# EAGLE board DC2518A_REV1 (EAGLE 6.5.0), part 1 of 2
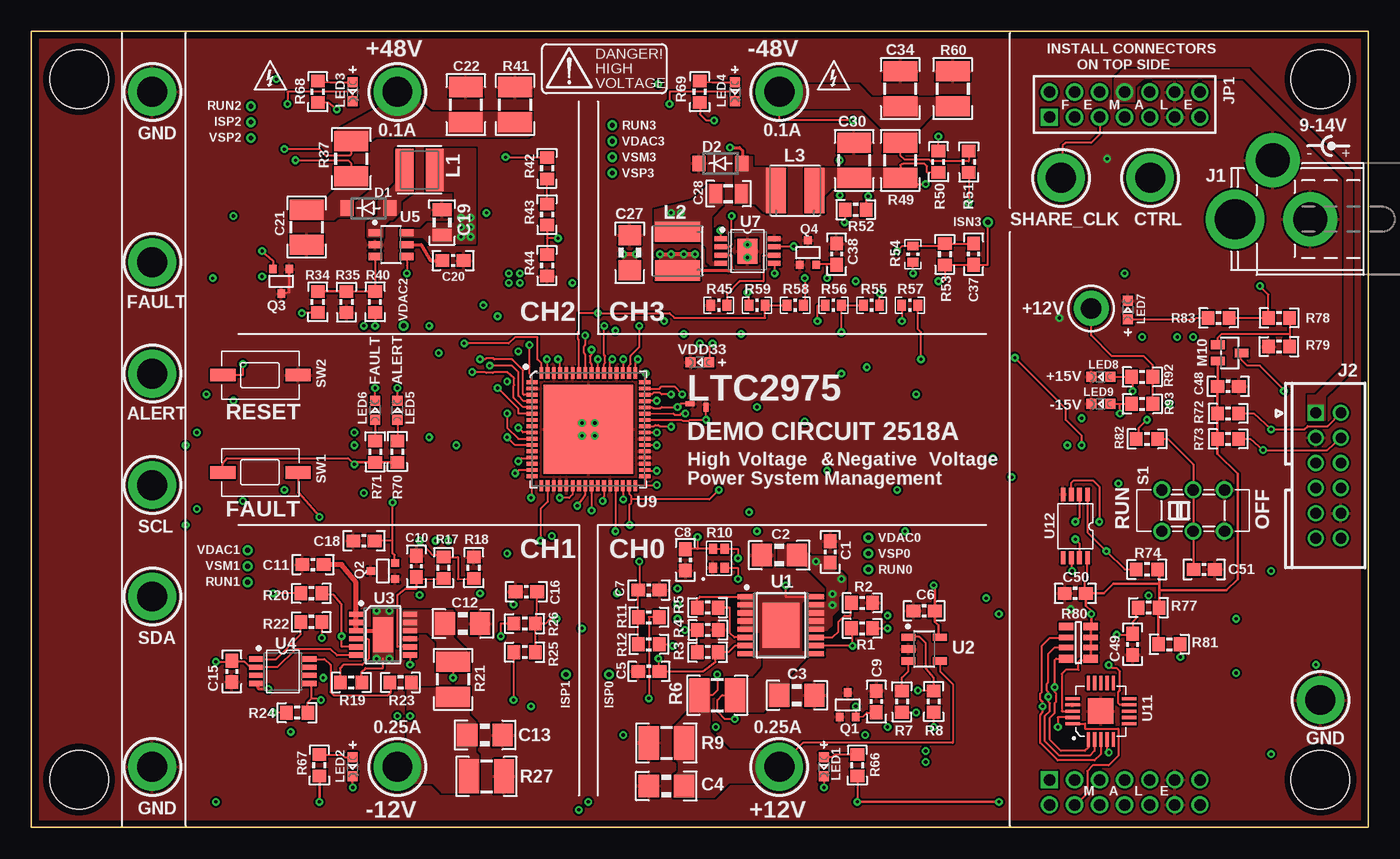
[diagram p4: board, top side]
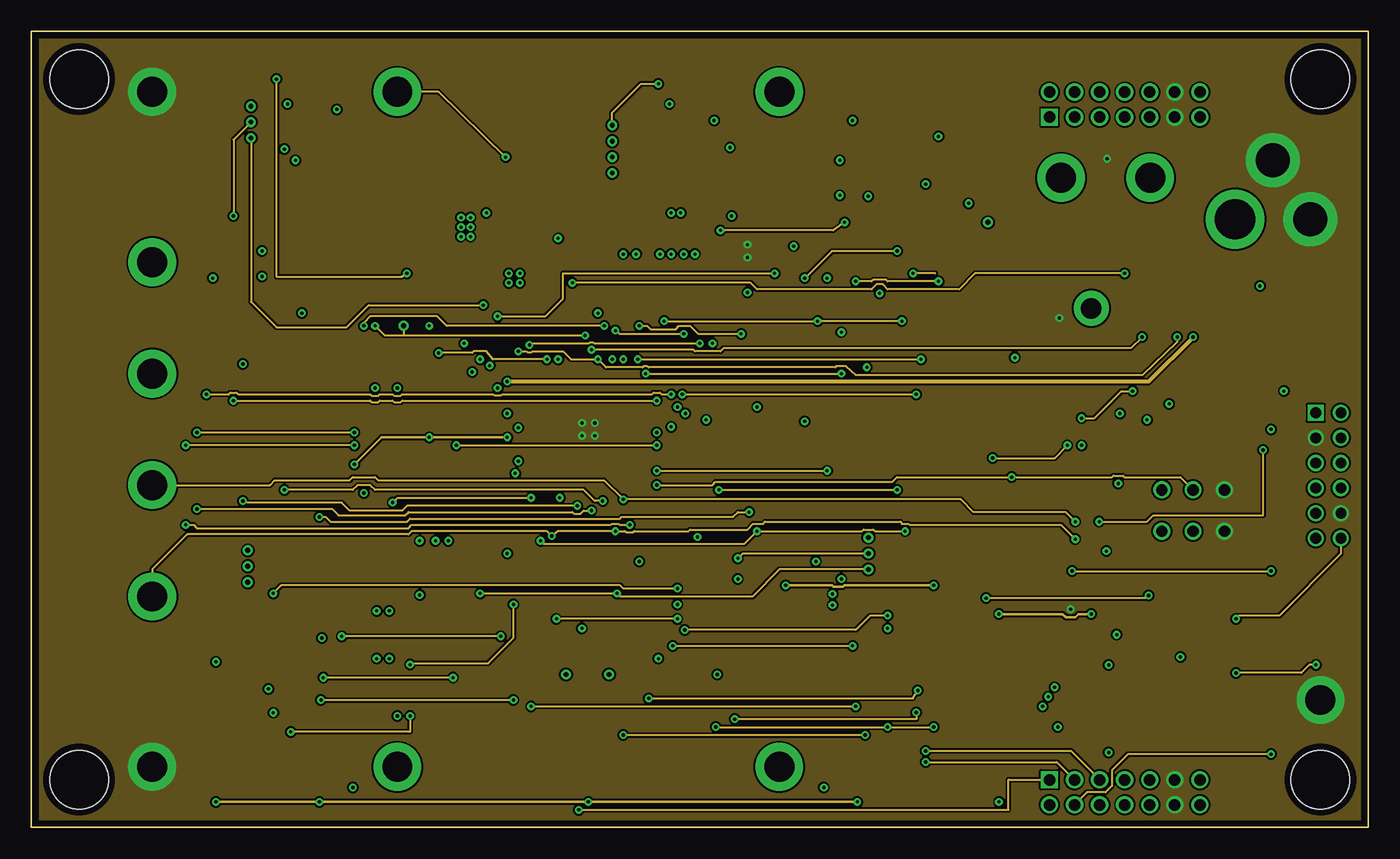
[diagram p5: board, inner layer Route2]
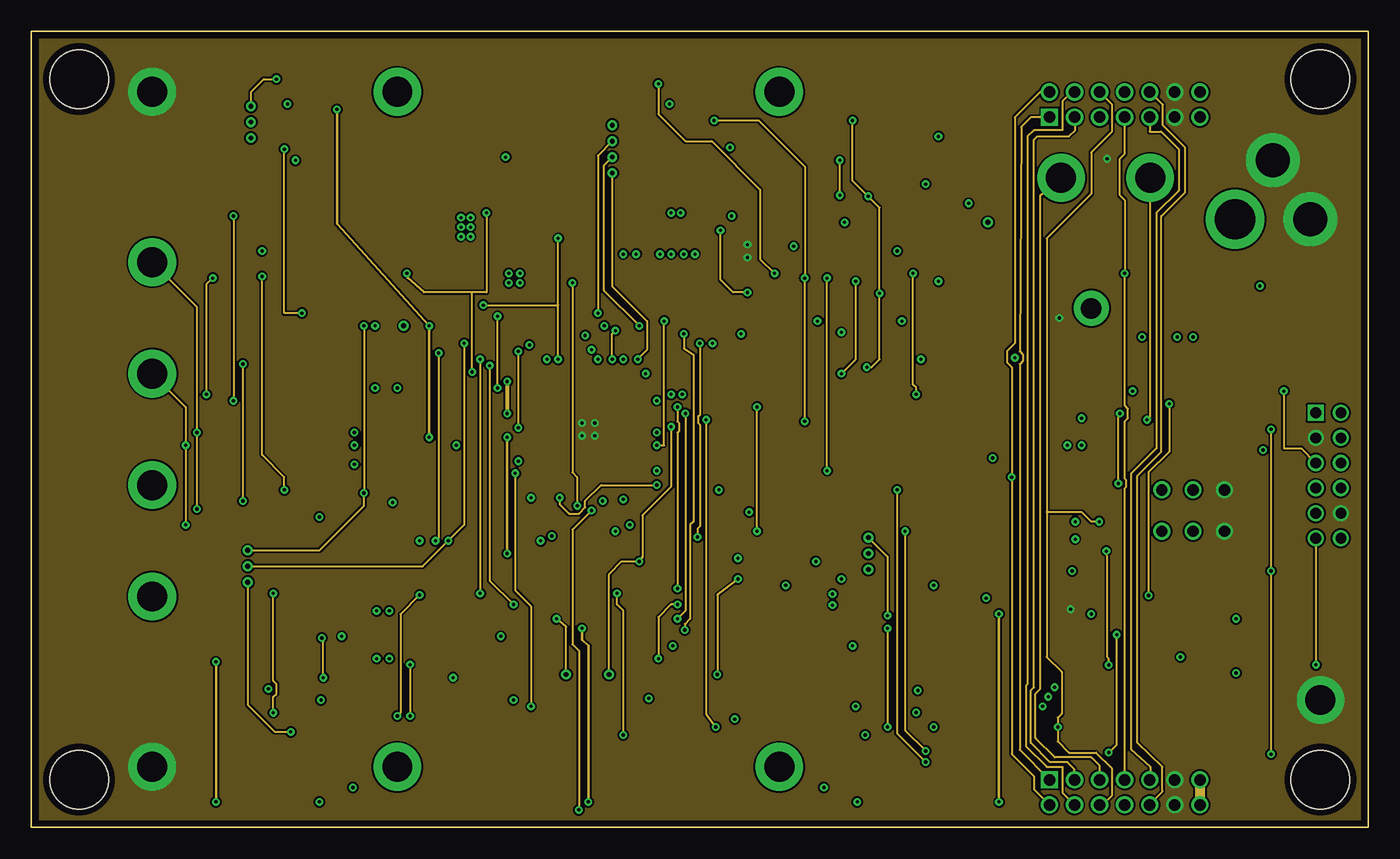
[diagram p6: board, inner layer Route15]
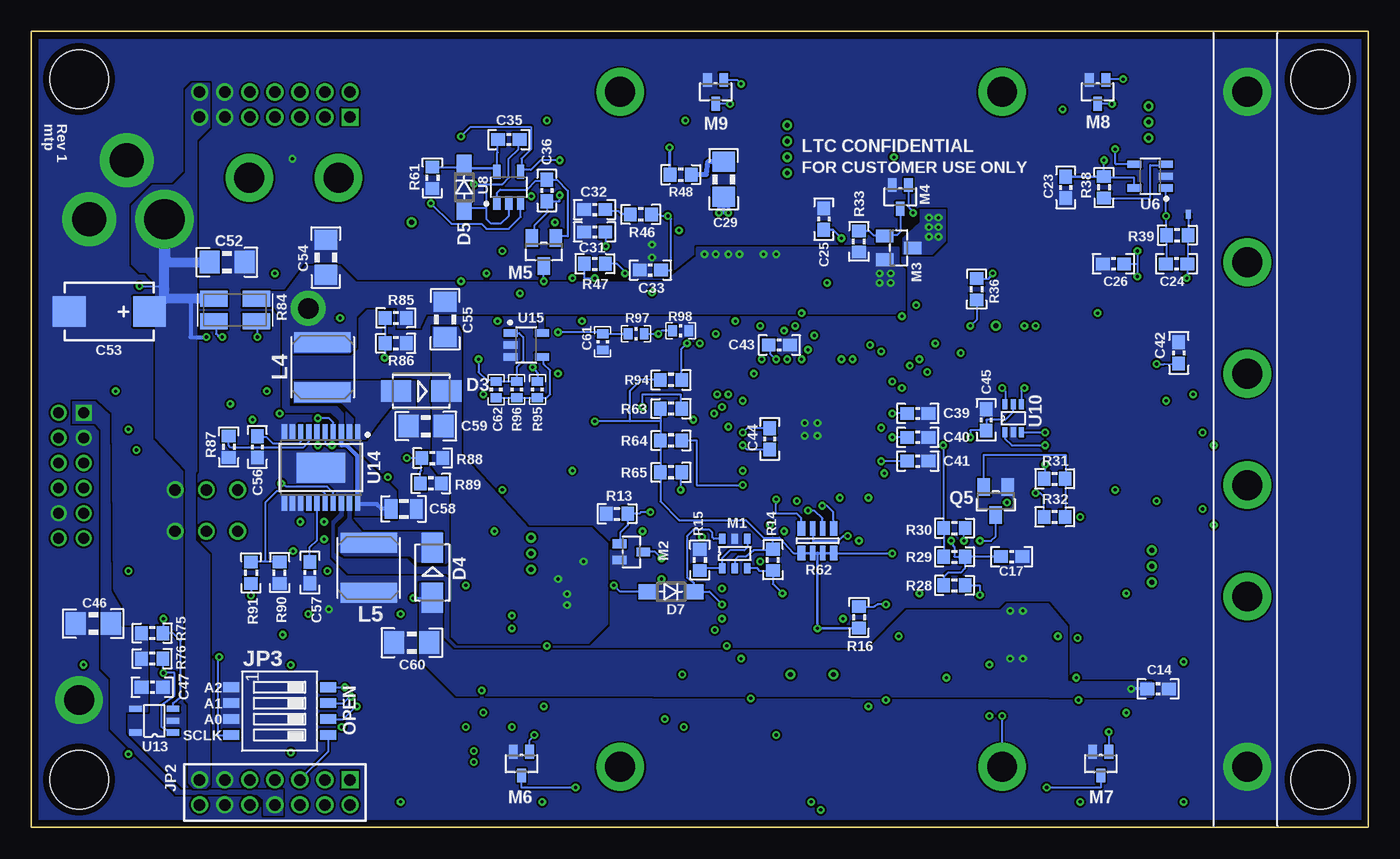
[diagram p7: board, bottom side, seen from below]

Size 106.68 x 63.5 mm. Coordinates in mm from the lower left corner, seen from the top.
Outline: 0,0 106.68,0 106.68,63.5 0,63.5 0,0
Copper layers (1*2+15*16): Top 0.06mm / dielectric 0.2mm / Route2 0.035mm / dielectric 1mm / Route15 0.035mm / dielectric 0.2mm / Bottom 0.06mm
Design rules "default *": minimum track width 6mil, minimum drill 10mil, track to track 6mil, track to pad 6mil, pad to pad 6mil, via to via 6mil, smd to smd 6mil, copper to edge 20mil, drill to drill 20mil, minimum pad ring 8mil, minimum via ring 7mil, stop-mask expansion 4mil, vias tented up to drill 14mil, thermal gap 6mil
Net classes: 1 HV: clearance 0.254 mm to class 0
Holes 4.7 mm at 3.81,3.81 102.87,3.81 3.81,59.69 102.87,59.69

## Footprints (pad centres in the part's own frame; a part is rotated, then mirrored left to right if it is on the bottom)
C0603_BOX = smd 1.1 x 1: 1 -0.85,0; 2 0.85,0
C1206_BOX = smd 1.6 x 1.8: 1 -1.4,0; 2 1.4,0
C0805_BOX = smd 1.016 x 1.524: 1 -1.016,0; 2 1.016,0
C1210_BOX = smd 1.6 x 2.7: 1 -1.4,0; 2 1.4,0
C7343 = smd 2.6 x 2.4: + -3.2,0; - 3.2,0
C0402_BOX = smd 0.7 x 0.9: 1 -0.65,0; 2 0.65,0
SOD123FL = smd 1.04 x 1.22: A 1.72,0; C -1.72,0
SMA = smd 2.4 x 1.7: A 2,0; C -2,0
SOD123 = smd 1.4 x 1.2: A 1.9,0; C -1.9,0
PJ-002A = drill 3.2 pad 4.7: 1 3,0 | drill 2.7 pad 4.3: 2 -3,0; 3 0,-4.7
CONN_DC1613 = drill 0.86 square: 1 -5,-1 | drill 0.86: 2 -5,1; 3 -3,-1; 4 -3,1; 5 -1,-1; 6 -1,1; 7 1,-1; 8 1,1; 9 3,-1; 10 3,1; 11 5,-1; 12 5,1
2X07M = drill 0.914 square: 1 -6,-1 | drill 0.914: 2 -6,1; 3 -4,-1; 4 -4,1; 5 -2,-1; 6 -2,1; 7 0,-1; 8 0,1; 9 2,-1; 10 2,1; 11 4,-1; 12 4,1; 13 6,-1; 14 6,1
SMT_DIP_4 = smd 1.27 x 0.762: 1 -3.861,1.905; 2 -3.861,0.635; 3 -3.861,-0.635; 4 -3.861,-1.905; 5 3.861,-1.905; 6 3.861,-0.635; 7 3.861,0.635; 8 3.861,1.905
WE-MAPI-3015 = smd 1.4 x 3.4: 1 -1.2,0; 2 1.2,0
WE-LQS-4018 = smd 1.6 x 3.6: 1 -1.55,0; 2 1.55,0
WE-LQS-5040 = smd 1.6 x 4.5: 1 -2,0; 2 2,0
0603 = smd 0.8 x 0.8: A 0,-0.75; C 0,0.75
TSOP-6 = smd 0.8 x 0.5: 1 -1.163,1; 2 -1.163,0; 3 -1.163,-1; 4 1.163,-1; 5 1.163,0; 6 1.163,1
SOT323 = smd 0.7 x 1.1: 1 -0.65,-0.95; 2 0.65,-0.95; 3 0,0.95
SOT23 = smd 1 x 1.4: 1 -0.95,-1.1; 2 0.95,-1.1; 3 0,1.1
SC70 = smd 0.6 x 0.65: 1 -0.65,-0.975; 2 0.65,-0.975; 3 0,0.975
R0603_BOX = smd 1 x 1.1: 1 -0.85,0; 2 0.85,0
R1210_BOX = smd 1.6 x 2.7: 1 -1.4,0; 2 1.4,0
R_ARRAY_2X_ACAS = smd 0.64 x 0.8: P$1 -0.47,-0.75; P$2 0.47,-0.75; P$3 0.47,0.75; P$4 -0.47,0.75
R0402_BOX = smd 0.7 x 0.9: 1 -0.65,0; 2 0.65,0
R_VISHAY_CRA06S = smd 1.15 x 0.63: R1_1 -0.975,1.295; R1_2 0.975,1.295; R4_1 -0.975,-1.295; R4_2 0.975,-1.295 | smd 1.15 x 0.44: R2_1 -0.975,0.4; R2_2 0.975,0.4; R3_1 -0.975,-0.4; R3_2 0.975,-0.4
LVK20 = smd 1.3 x 2.2: E1 0.9,-1.7; E2 0.9,1.7; I1 -0.9,-1.7; I2 -0.9,1.7
6-DPDT = drill 0.9: 1 -2.5,1.65; 2 0,1.65; 3 2.5,1.65; 4 -2.5,-1.65; 5 0,-1.65; 6 2.5,-1.65
SWITCH_PTS635 = smd 2 x 1: SW1 -3,0; SW2 3,0
TURRET_LARGE_2501 = drill 2.388 pad 3.81: TP 0,0
TURRET_SMALL_2308 = drill 1.626 pad 2.794: TP1 0,0
VIA = drill 0.381: 1 0,0
TSSOP16EXP = smd 0.42 x 1.2: 1 -2.275,-2.85; 2 -1.625,-2.85; 3 -0.975,-2.85; 4 -0.325,-2.85; 5 0.325,-2.85; 6 0.975,-2.85; 7 1.625,-2.85; 8 2.275,-2.85; 9 2.275,2.85; 10 1.625,2.85; 11 0.975,2.85; 12 0.325,2.85; 13 -0.325,2.85; 14 -0.975,2.85; 15 -1.625,2.85; 16 -2.275,2.85 | smd 3.58 x 2.94: EXP 0,0
TSOT23-5 = smd 0.58 x 1.1: 1 -0.95,-1.25; 2 0,-1.25; 3 0.95,-1.25; 4 0.95,1.25; 5 -0.95,1.25
MSOP12_EXP = smd 1.1 x 0.42: 1 -2.15,1.625; 2 -2.15,0.975; 3 -2.15,0.325; 4 -2.15,-0.325; 5 -2.15,-0.975; 6 -2.15,-1.625; 7 2.15,-1.625; 8 2.15,-0.975; 9 2.15,-0.325; 10 2.15,0.325; 11 2.15,0.975; 12 2.15,1.625 | smd 1.6 x 2.8: PAD 0,0
MSOP8 = smd 0.42 x 1.1: 1 -0.98,-2.15; 2 -0.33,-2.15; 3 0.32,-2.15; 4 0.97,-2.15; 5 0.97,2.15; 6 0.32,2.15; 7 -0.33,2.15; 8 -0.98,2.15
TSOT23-6 = smd 0.58 x 1.1: 1 -0.95,-1.25; 2 0,-1.25; 3 0.95,-1.25; 4 0.95,1.25; 5 0,1.25; 6 -0.95,1.25
MSOP8_EXP = smd 0.4 x 1: 1 -0.975,-2.15; 2 -0.325,-2.15; 3 0.325,-2.15; 4 0.975,-2.15; 5 0.975,2.15; 6 0.325,2.15; 7 -0.325,2.15; 8 -0.975,2.15 | smd 2 x 1.6: PAD 0,0
QFN64_9X9 = smd 0.9 x 0.3: 1 -4.5,3.75; 2 -4.5,3.25; 3 -4.5,2.75; 4 -4.5,2.25; 5 -4.5,1.75; 6 -4.5,1.25; 7 -4.5,0.75; 8 -4.5,0.25; 9 -4.5,-0.25; 10 -4.5,-0.75; 11 -4.5,-1.25; 12 -4.5,-1.75; 13 -4.5,-2.25; 14 -4.5,-2.75; 15 -4.5,-3.25; 16 -4.5,-3.75; 33 4.5,-3.75; 34 4.5,-3.25; 35 4.5,-2.75; 36 4.5,-2.25; 37 4.5,-1.75; 38 4.5,-1.25; 39 4.5,-0.75; 40 4.5,-0.25; 41 4.5,0.25; 42 4.5,0.75; 43 4.5,1.25; 44 4.5,1.75; 45 4.5,2.25; 46 4.5,2.75; 47 4.5,3.25; 48 4.5,3.75 | smd 0.3 x 0.9: 17 -3.75,-4.5; 18 -3.25,-4.5; 19 -2.75,-4.5; 20 -2.25,-4.5; 21 -1.75,-4.5; 22 -1.25,-4.5; 23 -0.75,-4.5; 24 -0.25,-4.5; 25 0.25,-4.5; 26 0.75,-4.5; 27 1.25,-4.5; 28 1.75,-4.5; 29 2.25,-4.5; 30 2.75,-4.5; 31 3.25,-4.5; 32 3.75,-4.5; 49 3.75,4.5; 50 3.25,4.5; 51 2.75,4.5; 52 2.25,4.5; 53 1.75,4.5; 54 1.25,4.5; 55 0.75,4.5; 56 0.25,4.5; 57 -0.25,4.5; 58 -0.75,4.5; 59 -1.25,4.5; 60 -1.75,4.5; 61 -2.25,4.5; 62 -2.75,4.5; 63 -3.25,4.5; 64 -3.75,4.5 | smd 7.112 x 7.112: PAD 0,0
SC70-6 = smd 0.4 x 0.8: 1 -0.65,-1.102; 2 0,-1.102; 3 0.65,-1.102; 4 0.65,1.102; 5 0,1.098; 6 -0.65,1.102
QFN20 = smd 1.143 x 0.254: 1 -2.25,1; 2 -2.25,0.5; 3 -2.25,0; 4 -2.25,-0.5; 5 -2.25,-1; 11 2.25,-1; 12 2.25,-0.5; 13 2.25,0; 14 2.25,0.5; 15 2.25,1 | smd 0.254 x 1.143: 6 -1,-2.25; 7 -0.5,-2.25; 8 0,-2.25; 9 0.5,-2.25; 10 1,-2.25; 16 1,2.25; 17 0.5,2.25; 18 0,2.25; 19 -0.5,2.25; 20 -1,2.25 | smd 2.032 x 2.032: PAD 0,0
MSOP-8 = smd 1.041 x 0.381: 1 -2.55,0.975; 2 -2.55,0.325; 3 -2.55,-0.325; 4 -2.55,-0.975; 5 2.479,-0.975; 6 2.479,-0.325; 7 2.479,0.325; 8 2.479,0.975
SOT-23-5 = smd 1 x 0.5: 1 -1.649,0.95; 2 -1.649,0; 3 -1.649,-0.95; 4 1.333,-0.95; 5 1.333,0.95
TSSOP20EXP = smd 0.42 x 1.2: 1 -2.925,-2.85; 2 -2.275,-2.85; 3 -1.625,-2.85; 4 -0.975,-2.85; 5 -0.325,-2.85; 6 0.325,-2.85; 7 0.975,-2.85; 8 1.625,-2.85; 9 2.275,-2.85; 10 2.925,-2.85; 11 2.925,2.85; 12 2.275,2.85; 13 1.625,2.85; 14 0.975,2.85; 15 0.325,2.85; 16 -0.325,2.85; 17 -0.975,2.85; 18 -1.625,2.85; 19 -2.275,2.85; 20 -2.925,2.85 | smd 3.86 x 2.4: EXP 0,0
KELVIN = smd 0.33 x 0.406: P$1 0.191,0; P$2 -0.191,0

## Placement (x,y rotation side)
C1  0.1uF  [C0603_BOX]  63.75,21.97 90 top
C2  10uF  [C1206_BOX]  59.69,21.72 180 top
C3  10uF/25V  [C1206_BOX]  61.09,10.54 0 top
C4  10uF/25V  [C1206_BOX]  50.67,3.3 180 top
C5  22nF  [C0603_BOX]  49.28,12.45 180 top
C6  0.1uF  [C0603_BOX]  71.25,17.27 180 top
C7  22nF  [C0603_BOX]  49.28,18.92 0 top
C8  10nF  [C0603_BOX]  52.2,21.34 270 top
C9  0.1uF  [C0603_BOX]  67.44,10.03 90 top
C10  22nF  [C0603_BOX]  30.73,20.83 270 top
C11  0.1uF  [C0603_BOX]  22.48,20.95 180 top
C12  4.7uF  [C1206_BOX]  34.42,16.26 0 top
C13  4.7uF  [C1206_BOX]  36.2,7.37 0 top
C14  0.1uF  [C0603_BOX]  16.76,11.05 0 bottom
C15  0.1uF  [C0603_BOX]  16,12.45 270 top
C16  47nF  [C0603_BOX]  39.5,18.8 180 top
C17  10nF  [C0603_BOX]  28.45,21.59 0 bottom
C18  0.1uF  [C0603_BOX]  26.54,22.86 180 top
C19  4.7uF/25V  [C0805_BOX]  32.77,48.26 90 top
C20  1uF  [C0603_BOX]  33.66,45.21 0 top
C21  2.2uF/100V  [C1210_BOX]  21.97,47.88 270 top
C22  2.2uF/100V  [C1210_BOX]  34.67,57.66 90 top
C23  0.1uF/100V  [C0603_BOX]  24.13,51.05 270 bottom
C24  47nF  [C0603_BOX]  15.29,44.96 0 bottom
C25  10nF  [C0603_BOX]  43.43,48.51 90 bottom
C26  0.1uF  [C0603_BOX]  20.32,44.96 180 bottom
C27  4.7uF/25V  [C1206_BOX]  47.75,45.85 90 top
C28  1uF/100V  [C0805_BOX]  55.63,50.55 0 top
C29  2.2uF/100V  [C1206_BOX]  51.44,51.69 270 bottom
C30  2.2uF/100V  [C1210_BOX]  65.66,53.21 90 top
C31  47nF  [C0603_BOX]  61.72,47.5 180 bottom
C32  1nF  [C0603_BOX]  61.72,49.28 180 bottom
C33  47pF  [C0603_BOX]  57.28,44.45 180 bottom
C34  2.2uF/100V  [C1210_BOX]  69.34,58.93 270 top
C35  0.1uF  [C0603_BOX]  68.58,54.86 0 bottom
C36  10nF  [C0603_BOX]  65.53,50.8 90 bottom
C37  47nF  [C0603_BOX]  75.18,45.72 270 top
C38  0.1uF  [C0603_BOX]  64.26,45.72 90 top
C39  0.1uF  [C0603_BOX]  35.94,33.02 0 bottom
C40  0.1uF  [C0603_BOX]  35.94,31.11 0 bottom
C41  0.1uF  [C0603_BOX]  35.94,29.21 0 bottom
C42  10nF  [C0603_BOX]  15.11,37.85 90 bottom
C43  0.1uF  [C0603_BOX]  46.99,38.48 0 bottom
C44  0.1uF  [C0603_BOX]  47.75,30.99 270 bottom
C45  0.1uF  [C0603_BOX]  30.48,32.51 90 bottom
C46  4.7uF/10V  [C1206_BOX]  101.73,16.26 180 bottom
C47  0.1uF  [C0603_BOX]  97.03,11.18 0 bottom
C48  0.1uF  [C0603_BOX]  95.5,35.18 0 top
C49  1uF  [C0603_BOX]  87.88,14.61 270 top
C50  0.1uF  [C0603_BOX]  83.31,18.67 180 top
C51  1uF  [C0603_BOX]  93.6,20.57 0 top
C52  10uF/25V  [C1206_BOX]  91.06,45.09 180 bottom
C53  47uF/16V  [C7343]  100.46,41.15 180 bottom
C54  2.2uF/25V  [C1206_BOX]  83.19,45.47 90 bottom
C55  1uF/25V  [C1206_BOX]  73.66,40.51 270 bottom
C56  47nF  [C0603_BOX]  88.65,30.35 270 bottom
C57  47nF  [C0603_BOX]  84.45,20.32 270 bottom
C58  1uF/25V  [C0805_BOX]  76.96,25.4 180 bottom
C59  22uF/25V  [C1206_BOX]  75.18,32 180 bottom
C60  22uF/25V  [C1206_BOX]  76.33,14.73 0 bottom
C61  47nF  [C0402_BOX]  61.09,38.73 270 bottom
C62  10nF  [C0402_BOX]  69.6,34.92 270 bottom
D1  MBR0580  [SOD123FL]  26.92,49.4 0 top
D2  MBR0580  [SOD123FL]  54.99,52.96 0 top
D3  B140-13-F  [SMA]  75.56,34.8 180 bottom
D4  B140-13-F  [SMA]  74.68,20.32 270 bottom
D5  5.6V  [SOD123]  72.14,51.05 270 bottom
D7  [SOD123]  55.63,18.8 180 bottom
J1  PJ-002A  [PJ-002A]  99.06,48.51 180 top
J2  CONN_DC1613  [CONN_DC1613]  103.5,28.07 270 top
JP1  FEMALE  [2X07M]  87.25,57.66 0 top
JP2  MALE  [2X07M]  87.25,2.79 180 bottom
JP3  TDA04H0SK1  [SMT_DIP_4]  86.87,9.27 0 bottom
L1  10uH  [WE-MAPI-3015]  30.99,52.45 180 top
L2  47uH  [WE-LQS-4018]  51.56,45.97 90 top
L3  100uH  [WE-LQS-4018]  60.96,50.8 0 top
L4  6.8uH  [WE-LQS-5040]  83.44,36.7 270 bottom
L5  10uH  [WE-LQS-5040]  79.76,20.7 90 bottom
LED1  GREEN  [0603]  63.25,4.83 180 top
LED2  GREEN  [0603]  25.65,4.83 180 top
LED3  GREEN  [0603]  25.65,58.67 180 top
LED4  GREEN  [0603]  56.13,58.67 180 top
LED5  RED  [0603]  29.21,33.27 0 top
LED6  RED  [0603]  27.43,33.27 0 top
LED7  BLUE  [0603]  87.5,41.27 0 top
LED8  BLUE  [0603]  85.34,35.94 90 top
LED9  BLUE  [0603]  85.34,33.78 90 top
LED10  GREEN  [0603]  53.34,37.08 90 top
M1  Si3552DV  [TSOP-6]  50.55,21.84 90 bottom
M2  DMG1012  [SOT323]  58.8,21.97 270 bottom
M3  DMP3098L  [SOT23]  37.47,46.23 270 bottom
M4  DMG1012  [SOT323]  37.34,50.29 180 bottom
M5  ZVN3310  [SOT23]  65.79,45.9 180 bottom
M6  DMG1012  [SOT323]  67.56,5.08 180 bottom
M7  DMG1012  [SOT323]  21.34,5.08 180 bottom
M8  DMG1012  [SOT323]  21.59,58.67 180 bottom
M9  DMG1012  [SOT323]  52.07,58.67 180 bottom
M10  NTS4173P  [SOT323]  95.63,37.85 270 top
Q1  MMST3906  [SC70]  65.15,9.78 0 top
Q2  MMST3906  [SC70]  28.07,20.45 90 top
Q3  MMST3906  [SC70]  19.94,43.56 180 top
Q4  MMST3906  [SC70]  61.98,45.85 0 top
Q5  2N3906  [SOT23]  29.72,26.04 180 bottom
R1  2.0k  [R0603_BOX]  66.29,15.88 0 top
R2  1k  [R0603_BOX]  66.29,17.91 0 top
R3  215k  [R0603_BOX]  53.98,13.97 180 top
R4  24.9k  [R0603_BOX]  53.98,15.75 0 top
R5  1.5k  [R0603_BOX]  53.98,17.53 180 top
R6  50m  [R1210_BOX]  54.74,10.54 180 top
R7  100  [R0603_BOX]  69.47,10.03 90 top
R8  1.0k  [R0603_BOX]  72.01,10.03 270 top
R9  2.0k  [R1210_BOX]  50.67,6.73 180 top
R10  1k,2k Array  [R_ARRAY_2X_ACAS]  54.86,21.46 0 top
R11  0R  [R0603_BOX]  49.28,16.76 0 top
R12  0R  [R0603_BOX]  49.28,14.61 0 top
R13  100k  [R0603_BOX]  59.94,25.02 0 bottom
R14  10k  [R0603_BOX]  47.5,21.34 270 bottom
R15  10k  [R0603_BOX]  53.34,21.34 90 bottom
R16  10k  [R0603_BOX]  40.64,16.76 90 bottom
R17  200k  [R0603_BOX]  32.89,20.7 270 top
R18  69.8k  [R0603_BOX]  35.31,20.7 270 top
R19  20k  [R0603_BOX]  25.53,11.56 0 top
R20  1k  [R0603_BOX]  22.35,18.67 180 top
R21  50m  [R1210_BOX]  33.66,11.81 270 top
R22  100  [R0603_BOX]  22.35,16.38 180 top
R23  100  [R0603_BOX]  29.46,11.56 180 top
R24  1.0k  [R0603_BOX]  21.21,9.14 180 top
R25  0R  [R0603_BOX]  39.37,13.97 180 top
R26  0R  [R0603_BOX]  39.37,16.26 180 top
R27  1.21k  [R1210_BOX]  36.32,4.06 0 top
R28  140k  [R0603_BOX]  33.02,19.3 0 bottom
R29  10k  [R0603_BOX]  33.02,21.59 0 bottom
R30  0  [R0603_BOX]  33.02,23.88 0 bottom
R31  130k  [R0603_BOX]  25.02,27.81 0 bottom
R32  40.2k  [R0603_BOX]  25.02,24.77 0 bottom
R33  10k  [R0603_BOX]  40.64,46.74 270 bottom
R34  294k  [R0603_BOX]  22.86,41.91 270 top
R35  10.0k  [R0603_BOX]  25.15,41.91 90 top
R36  10k  [R0603_BOX]  31.24,42.93 270 bottom
R37  50m  [R1210_BOX]  25.53,53.34 90 top
R38  100  [R0603_BOX]  21.08,51.05 90 bottom
R39  2.0k  [R0603_BOX]  15.24,47.24 0 bottom
R40  90.9k  [R0603_BOX]  27.43,41.91 270 top
R41  13.7k  [R1210_BOX]  38.61,57.66 90 top
R42  13.7k  [R0603_BOX]  41.15,52.58 90 top
R43  13.3k  [R0603_BOX]  41.15,48.9 90 top
R44  3.01k  [R0603_BOX]  41.15,44.83 90 top
R45  46.4k  [R0402_BOX]  54.86,41.66 180 top
R46  14k  [R0603_BOX]  58.04,48.9 180 bottom
R47  10k  [R0603_BOX]  61.72,44.96 0 bottom
R48  49.9  [R0603_BOX]  54.86,52.07 0 bottom
R49  50m  [R1210_BOX]  69.34,53.21 90 top
R50  100  [R0603_BOX]  72.39,53.09 270 top
R51  100  [R0603_BOX]  74.8,53.09 90 top
R52  464k  [R0603_BOX]  65.79,49.28 0 top
R53  2.0k  [R0603_BOX]  72.9,45.72 90 top
R54  0  [R0402_BOX]  70.36,45.72 90 top
R55  953k  [R0402_BOX]  67.06,41.66 0 top
R56  16.2k  [R0402_BOX]  64.01,41.66 0 top
R57  0  [R0402_BOX]  70.1,41.66 0 top
R58  133k  [R0402_BOX]  60.96,41.66 0 top
R59  33.2k  [R0402_BOX]  57.91,41.66 0 top
R60  9.76k  [R1210_BOX]  73.53,58.93 90 top
R61  40.2k  [R0603_BOX]  74.68,51.82 90 bottom
R62  10k (x4)  [R_VISHAY_CRA06S]  43.94,22.86 270 bottom
R63  10k  [R0603_BOX]  55.63,33.4 180 bottom
R64  10k  [R0603_BOX]  55.63,30.86 180 bottom
R65  10k  [R0603_BOX]  55.63,28.32 180 bottom
R66  10k  [R0603_BOX]  65.91,4.95 270 top
R67  10k  [R0603_BOX]  22.99,4.95 270 top
R68  10k  [R0603_BOX]  22.86,58.67 270 top
R69  10k  [R0603_BOX]  53.34,58.67 270 top
R70  1k  [R0603_BOX]  29.21,29.97 270 top
R71  1k  [R0603_BOX]  27.43,29.97 90 top
R72  10k  [R0603_BOX]  95.5,33.02 0 top
R73  10k  [R0603_BOX]  95.5,30.99 0 top
R74  10k  [R0603_BOX]  89.03,20.57 180 top
R75  10k  [R0603_BOX]  97.03,15.49 180 bottom
R76  10k  [R0603_BOX]  97.03,13.46 180 bottom
R77  249  [R0603_BOX]  89.15,17.53 180 top
R78  100k  [R0603_BOX]  99.57,40.64 0 top
R79  100k  [R0603_BOX]  99.57,38.35 180 top
R80  10k (x4)  [R_VISHAY_CRA06S]  83.57,14.73 0 top
R81  10k  [R0603_BOX]  90.81,14.61 0 top
R82  10k  [R0603_BOX]  89.03,30.99 0 top
R83  30k  [R0603_BOX]  94.74,40.64 0 top
R84  10m  [LVK20]  90.42,41.27 270 bottom
R85  80.6k  [R0603_BOX]  77.6,40.64 0 bottom
R86  16.5k  [R0603_BOX]  77.6,38.61 180 bottom
R87  130k  [R0603_BOX]  90.93,30.35 90 bottom
R88  182k  [R0603_BOX]  74.68,29.46 0 bottom
R89  10k  [R0603_BOX]  74.8,27.43 180 bottom
R90  10k  [R0603_BOX]  86.87,20.32 270 bottom
R91  182k  [R0603_BOX]  89.15,20.32 90 bottom
R92  30k  [R0603_BOX]  88.65,35.94 0 top
R93  30k  [R0603_BOX]  88.65,33.78 0 top
R94  10k  [R0603_BOX]  55.63,35.69 180 bottom
R95  100k  [R0402_BOX]  66.29,34.92 270 bottom
R96  10k  [R0402_BOX]  67.94,34.92 270 bottom
R97  0  [R0402_BOX]  58.42,39.37 0 bottom
R98  0  [R0402_BOX]  54.86,39.62 0 bottom
S1  JS202011CQN  [6-DPDT]  92.71,25.27 0 top
SW1  PTS635SL25SMTR LFS  [SWITCH_PTS635]  18.29,28.32 0 top
SW2  PTS635SL25SMTR LFS  [SWITCH_PTS635]  18.29,36.07 0 top
TP1  2501-2-00-80-00-00-07-0  [TURRET_LARGE_2501]  9.65,58.67 0 top
TP2  2501-2-00-80-00-00-07-0  [TURRET_LARGE_2501]  9.65,4.83 0 top
TP3  2501-2-00-80-00-00-07-0  [TURRET_LARGE_2501]  59.69,4.83 0 top
TP4  2501-2-00-80-00-00-07-0  [TURRET_LARGE_2501]  29.21,4.83 0 top
TP5  2501-2-00-80-00-00-07-0  [TURRET_LARGE_2501]  29.21,58.67 0 top
TP6  2501-2-00-80-00-00-07-0  [TURRET_LARGE_2501]  59.69,58.67 0 top
TP7  2501-2-00-80-00-00-07-0  [TURRET_LARGE_2501]  82.17,51.82 0 top
TP8  2501-2-00-80-00-00-07-0  [TURRET_LARGE_2501]  89.28,51.82 0 top
TP9  2501-2-00-80-00-00-07-0  [TURRET_LARGE_2501]  9.65,45.09 0 top
TP10  2501-2-00-80-00-00-07-0  [TURRET_LARGE_2501]  9.65,36.2 0 top
TP11  2501-2-00-80-00-00-07-0  [TURRET_LARGE_2501]  102.87,10.16 0 top
TP12  2501-2-00-80-00-00-07-0  [TURRET_LARGE_2501]  9.65,27.3 0 top
TP13  2501-2-00-80-00-00-07-0  [TURRET_LARGE_2501]  9.65,18.41 0 top
TP14  2308-2-00-80-00-00-07-0  [TURRET_SMALL_2308]  84.58,41.4 0 top
TP15  TESTPOINT  [VIA]  66.8,20.57 0 top
TP16  TESTPOINT  [VIA]  66.8,23.11 0 top
TP17  TESTPOINT  [VIA]  66.8,21.84 0 top
TP18  TESTPOINT  [VIA]  17.27,22.1 0 top
TP19  TESTPOINT  [VIA]  17.27,20.83 0 top
TP20  TESTPOINT  [VIA]  17.27,19.56 0 top
TP21  TESTPOINT  [VIA]  29.72,40.01 0 top
TP22  TESTPOINT  [VIA]  17.53,54.99 0 top
TP23  TESTPOINT  [VIA]  17.53,57.53 0 top
TP24  TESTPOINT  [VIA]  46.35,54.74 0 top
TP25  TESTPOINT  [VIA]  46.35,53.47 0 top
TP26  TESTPOINT  [VIA]  46.35,56.01 0 top
TP27  TESTPOINT  [VIA]  46.1,12.19 0 top
TP28  TESTPOINT  [VIA]  42.67,12.19 0 top
TP29  TESTPOINT  [VIA]  17.53,56.26 0 top
TP30  TESTPOINT  [VIA]  76.33,48.26 0 top
TP31  TESTPOINT  [VIA]  46.35,52.2 0 top
U1  LT3081FE  [TSSOP16EXP]  59.82,16.13 270 top
U2  LTC6101  [TSOT23-5]  71.25,14.22 270 top
U3  LT3090MSE  [MSOP12_EXP]  28.07,15.37 0 top
U4  LT6105MS8  [MSOP8]  20.07,12.45 270 top
U5  LT8330  [TSOT23-6]  28.7,46.48 270 top
U6  LTC6101  [TSOT23-5]  17.4,51.94 90 bottom
U7  LT8580  [MSOP8_EXP]  57.15,45.97 270 top
U8  LTC2054  [TSOT23-5]  68.58,51.05 0 bottom
U9  LTC2975  [QFN64_9X9]  44.45,31.75 0 top
U10  SN74LVC2G34DCK  [SC70-6]  28.32,32.64 0 bottom
U11  MCP23008-E/ML  [QFN20]  85.34,9.27 90 top
U12  LTC4313CMS8  [MSOP-8]  83.31,24 270 top
U13  24AA02T-I/OT  [SOT-23-5]  97.03,8.51 180 bottom
U14  LT8471  [TSSOP20EXP]  83.57,28.7 180 bottom
U15  LT6015  [TSOT23-5]  67.18,38.48 270 bottom
U$20  [LT_LOGO_LARGE_SM]  5.33,10.16 90 top
U$21  [LT_LOGO_LARGE_SM]  2.03,10.16 90 bottom
U$32  [HV_SIGN_SMALL]  64.01,59.69 0 top
U$34  [HV_SIGN_SMALL]  19.05,59.69 0 top
U$35  [HV_SIGN]  45.97,60.71 0 top
U$38  [DC2518_FRAME]  not placed on the board
U$39  KELVIN-CONNECT  [KELVIN]  52.58,33.78 0 top
U$40  KELVIN-CONNECT  [KELVIN]  53.85,33.53 90 top
U$41  KELVIN-CONNECT  [KELVIN]  14.35,48.9 90 bottom
U$42  [DRILEGEND]  not placed on the board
